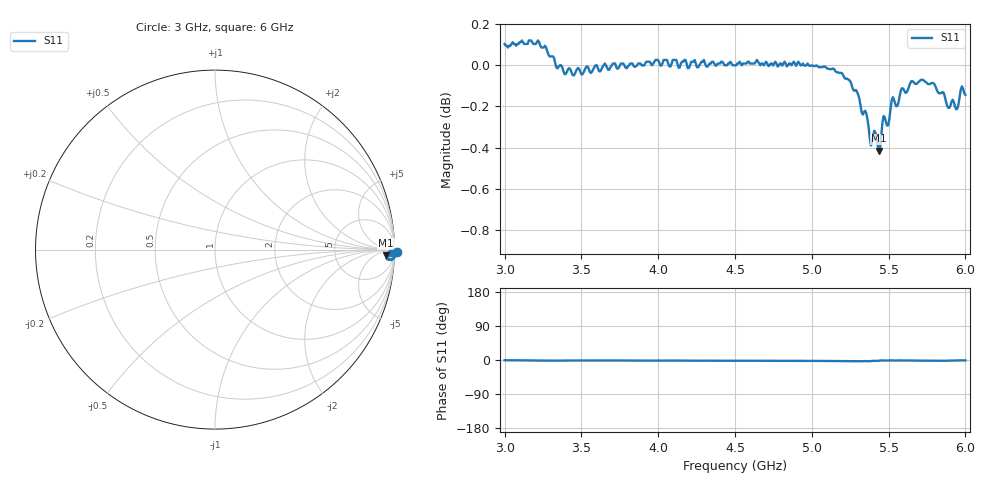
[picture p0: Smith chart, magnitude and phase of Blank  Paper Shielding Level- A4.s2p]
!  02/07/2025  16:02:05
! Ref Plane: 0.000 mm
# MHZ S MA R  50
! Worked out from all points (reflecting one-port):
!   401 points, 3 GHz to 6 GHz, reference 50 ohm
!   lowest |S11| = -0.4 dB at 5.438 GHz (marker M1), VSWR 41.83, Z = 1.43e+03 - j973 ohm
!   phase of S11 starts at -1 deg and turns -0 deg over the sweep
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3000  1.012 -0.7
3217.5  1.014 -1.4
3285  1.006 -1.7
3375  0.9991 -1.6
3450  0.9943 -1.4
3637.5  0.9991 -1.2
3750  0.9998 -1.3
4125  1.001 -1.7
4297.5  1.003 -2.0
4500  1 -2.0
4875  1.001 -2.2
5130  0.9979 -2.6
5250  0.9912 -3.1
5362.5  0.9703 -3.3
5385  0.9561 -2.8
5437.5  0.9533 -1.9
5452.5  0.9616 -1.1
5482.5  0.9688 -1.5
5512.5  0.9759 -0.8
5542.5  0.9788 -1.4
5572.5  0.9831 -1.0
5625  0.9862 -1.2
5715  0.992 -1.7
5812.5  0.9866 -2.0
5887.5  0.9766 -1.8
5940  0.9757 -1.3
5962.5  0.9824 -0.8
6000  0.9836 -1.0
